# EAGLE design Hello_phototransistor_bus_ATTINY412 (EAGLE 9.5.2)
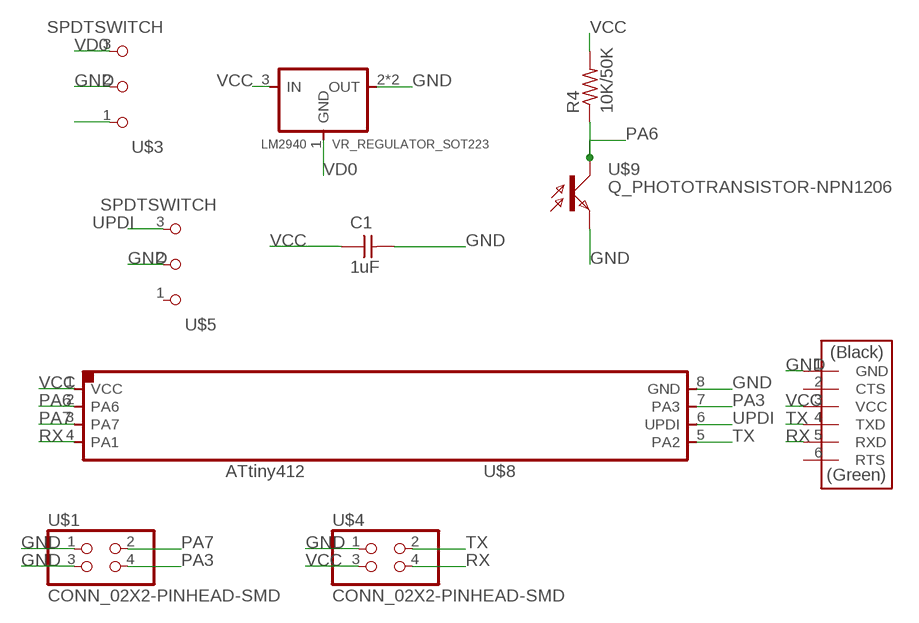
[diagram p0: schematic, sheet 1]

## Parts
C1  1uF  CAP_UNPOLARIZEDFAB  [C1206FAB]
LM2940  VR_REGULATOR_SOT223  [SOT223]
R4  10K/50K  R1206FAB  [R1206FAB]
U$1  CONN_02X2-PINHEAD-SMD  [2X02SMD]
U$2  CONN_06_FTDI-SMD-HEADER  [1X06SMD]
U$3  SPDTSWITCH  [SPDTSWITCH]
U$4  CONN_02X2-PINHEAD-SMD  [2X02SMD]
U$5  SPDTSWITCH  [SPDTSWITCH]
U$8  UC_ATTINY45SI  [SOIC8]
U$9  Q_PHOTOTRANSISTOR-NPN1206  [OP1206]

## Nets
GND: C1.2 LM2940.2(OUT) LM2940.4(OUT) U$1.1 U$1.3 U$2.1(GND) U$3.2 U$4.1 U$5.2 U$8.8(GND) U$9.EMITTER(E)
N$4: U$3.1
PA3: U$1.4 U$8.7(PA3)
PA6: R4.1 U$8.2(PA6) U$9.COLLECTOR(C)
PA7: U$1.2 U$8.3(PA7)
RX: U$2.5(RXD) U$4.4 U$8.4(PA1)
TX: U$2.4(TXD) U$4.2 U$8.5(PA2)
UPDI: U$5.3 U$8.6(UPDI)
VCC [New Class]: C1.1 LM2940.3(IN) R4.2 U$2.3(VCC) U$4.3 U$8.1(VCC)
VD0: LM2940.1(GND) U$3.3
Unconnected: U$2.2(CTS) U$2.6(RTS) U$5.1

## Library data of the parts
C1 = fab:CAP_UNPOLARIZED
LM2940 = fab:VR_REGULATOR_SOT223
R4 = fab:R: Resistor (US Symbol)
U$1 U$4 = fab:CONN_02X2-PINHEAD-SMD
U$2 = fab:CONN_06_FTDI-SMD-HEADER
U$3 U$5 = fab:SPDTSWITCH
U$8 = fab:UC_ATTINY45
U$9 = fab:Q_PHOTOTRANSISTOR-NPN

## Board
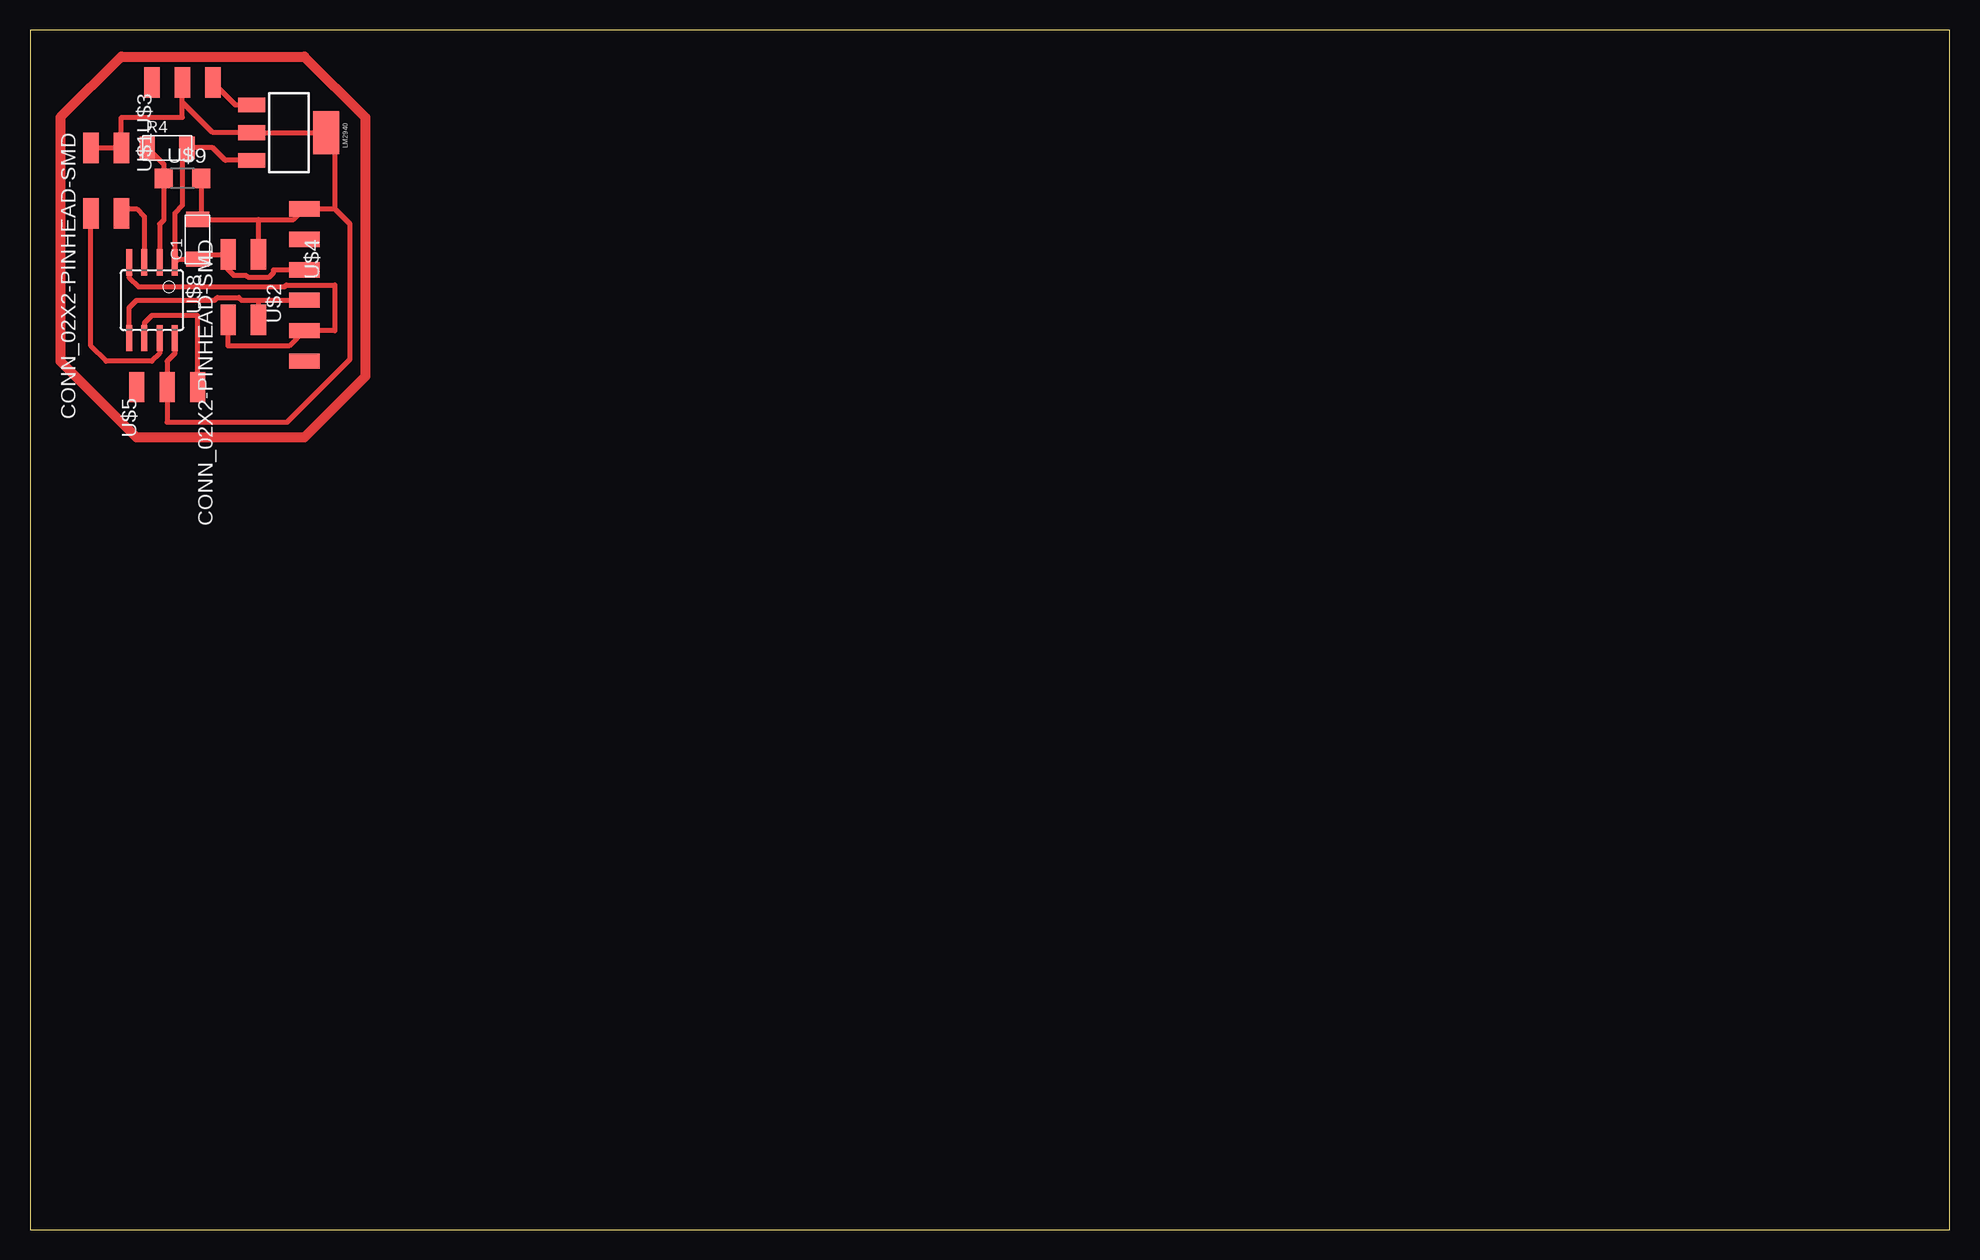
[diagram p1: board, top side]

Size 160 x 100 mm. Coordinates in mm from the lower left corner, seen from the top.
Outline: 0,0 160,0 160,100 0,100 0,0
Copper layers (1*16): Top 0.035mm / dielectric 1.5mm / Bottom 0.035mm
Design rules "default *": minimum track width 16mil, minimum drill 0.35mm, track to track 16mil, track to pad 16mil, pad to pad 16mil, via to via 16mil, smd to smd 6mil, copper to edge 40mil, drill to drill 6mil, minimum pad ring 10mil, minimum via ring 8mil, stop-mask expansion 4mil, vias tented up to drill 0mil, thermal gap 10mil

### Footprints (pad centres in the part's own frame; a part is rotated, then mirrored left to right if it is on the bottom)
C1206FAB = smd 1.27 x 1.905: 1 -1.651,0; 2 1.651,0
SOT223 = smd 1.219 x 2.235: 1 -2.311,-3.099; 2 0,-3.099; 3 2.311,-3.099 | smd 3.6 x 2.2: 4 0,3.099
R1206FAB = smd 1.27 x 1.905: 1 -1.651,0; 2 1.651,0
2X02SMD = smd 2.54 x 1.27: 1 -2.54,1.27; 2 2.92,1.27; 3 -2.54,-1.27; 4 2.92,-1.27
1X06SMD = smd 2.54 x 1.27: 1 0,6.35; 2 0,3.81; 3 0,1.27; 4 0,-1.27; 5 0,-3.81; 6 0,-6.35
SPDTSWITCH = smd 2.54 x 1.27: 1 0.38,2.54; 2 0.38,0; 3 0.38,-2.54
SOIC8 = smd 0.5 x 2.2: 1 -1.905,-3.154; 2 -0.645,-3.154; 3 0.625,-3.154; 4 1.895,-3.154; 5 1.905,3.154; 6 0.635,3.154; 7 -0.635,3.154; 8 -1.905,3.154
OP1206 = smd 1.5 x 1.6: COLLECTOR -1.55,0; EMITTER 1.55,0

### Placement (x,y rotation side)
C1  13.97,82.55 90 top
LM2940  21.59,91.44 270 top
R4  11.43,90.17 0 top
U$1  6.35,87.63 270 top
U$2  22.86,78.74 0 top
U$3  12.7,95.25 90 top
U$4  17.78,78.74 270 top
U$5  11.43,69.85 90 top
U$8  10.16,77.47 180 top
U$9  12.7,87.63 0 top

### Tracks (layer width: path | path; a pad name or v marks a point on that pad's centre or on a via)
GND
  Top 0.406: 19.05,84.2 C1.2 14.25,84.48 U$9.EMITTER | 19.05,84.2 21.97,84.2 U$2.1 25.4,85.09 | U$8.8 12.06,73.03 11.43,72.39 U$5.2 11.43,67.31 21.42,67.31 26.67,72.56 26.67,83.82 25.4,85.09 | U$4.1 19.05,84.2 | 25.4,85.09 25.4,90.73 LM2940.4 LM2940.2 15.24,91.44 12.7,93.98 | 12.7,93.98 U$3.2 | U$1.3 U$1.1 7.62,92.71 12.7,92.71 12.7,93.98
N$2
  Top 0.813: 7.62,97.79 22.86,97.79 27.94,92.71 27.94,71.12 22.86,66.04 8.89,66.04 2.54,72.39 2.54,92.71 7.62,97.79
PA3
  Top 0.406: U$8.7 10.79,73.03 10.16,72.39 6.35,72.39 5.08,73.66 U$1.4
PA6
  Top 0.406: U$8.2 10.8,83.82 11.15,84.17 U$9.COLLECTOR 11.15,88.8 R4.1
PA7
  Top 0.406: U$1.2 8,85.09 8.89,85.09 9.54,84.44 U$8.3
RX
  Top 0.406: U$8.4 8.27,79.36 9.04,78.59 21.21,78.59 21.36,78.74 25.4,78.74 25.4,74.93 U$2.5 21.59,73.66 16.51,73.66 U$4.4
TX
  Top 0.406: U$8.5 8.26,76.83 8.89,77.47 15.39,77.47 15.62,77.7 17.4,77.7 17.63,77.47 19.05,77.47 | U$4.2 19.05,77.47 | 19.05,77.47 U$2.4 21.59,77.47
UPDI
  Top 0.406: U$5.3 13.97,76.2 10.16,76.2 9.53,75.56 U$8.6
VCC
  Top 0.406: U$2.3 20.32,80.01 20.3,79.98 20.3,79.76 19.94,79.4 18.16,79.4 18.01,79.55 16.97,79.55 16.51,80.01 U$4.3 14.35,81.28 C1.1 12.34,80.9 U$8.1 12.06,84.75 12.7,85.38 12.7,89.79 R4.2 15.24,90.17 16.28,89.13 LM2940.3
VD0
  Top 0.406: U$3.3 17.12,93.75 LM2940.1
